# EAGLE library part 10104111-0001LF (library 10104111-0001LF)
FCI Right Angle SMT Female Type AB Version 2.0 Micro USB Connector, 100 V ac, 1.8A Source: Datasheet
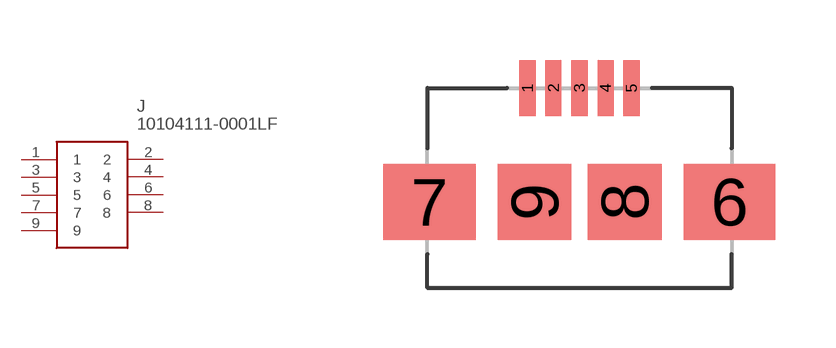
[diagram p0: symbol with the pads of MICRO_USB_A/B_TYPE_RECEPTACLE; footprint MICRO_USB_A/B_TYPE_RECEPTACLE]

Designator prefix J

## 10104111-0001LF (Allied_Number: 70236825; Description: FCI Right Angle SMT Female Type AB Version 2.0 Micro USB Connector, 100 V ac, 1.8A; Height: mm; Manufacturer_Name: FCI; Manufacturer_Part_Number: 10104111-0001LF; RS_Part_Number: 1622014)  [MICRO_USB_A/B_TYPE_RECEPTACLE]
1  1
2  2
3  3
4  4
5  5
6  6
7  7
8  8
9  9

## Footprint MICRO_USB_A/B_TYPE_RECEPTACLE (pad centres in mm)
MICRO_USB_A/B_TYPE_RECEPTACLE
smd 0.4 x 1.4: 1 2.5,5; 2 3.15,5; 3 3.8,5; 4 4.45,5; 5 5.1,5
smd 2.3 x 1.9: 6 7.55,2.15; 7 0.05,2.15
smd 1.85 x 1.9: 8 4.925,2.15; 9 2.675,2.15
